PROGRAM MAIN
VAR
	//  8_Slave  and 248Input word /248Output word
	wArrScanner2AdapterInput_1				AT%I*		:ARRAY[0..247] OF WORD;
	wArrAdapter2ScannerOutput_1				AT%Q*		:ARRAY[0..247] OF WORD;
	wArrScanner2AdapterInput_2				AT%I*		:ARRAY[0..247] OF WORD;
	wArrAdapter2ScannerOutput_2				AT%Q*		:ARRAY[0..247] OF WORD;
	wArrScanner2AdapterInput_3				AT%I*		:ARRAY[0..247] OF WORD;
	wArrAdapter2ScannerOutput_3				AT%Q*		:ARRAY[0..247] OF WORD;
	wArrScanner2AdapterInput_4				AT%I*		:ARRAY[0..247] OF WORD;
	wArrAdapter2ScannerOutput_4				AT%Q*		:ARRAY[0..247] OF WORD;
	wArrScanner2AdapterInput_5				AT%I*		:ARRAY[0..247] OF WORD;
	wArrAdapter2ScannerOutput_5				AT%Q*		:ARRAY[0..247] OF WORD;
	wArrScanner2AdapterInput_6				AT%I*		:ARRAY[0..247] OF WORD;
	wArrAdapter2ScannerOutput_6				AT%Q*		:ARRAY[0..247] OF WORD;
	wArrScanner2AdapterInput_7				AT%I*		:ARRAY[0..247] OF WORD;
	wArrAdapter2ScannerOutput_7				AT%Q*		:ARRAY[0..247] OF WORD;
	wArrScanner2AdapterInput_8				AT%I*		:ARRAY[0..247] OF WORD;
	wArrAdapter2ScannerOutput_8				AT%Q*		:ARRAY[0..247] OF WORD;
	i,j			:INT;
END_VAR

FOR i :=0 TO 247 DO
	wArrAdapter2ScannerOutput_1[i]			:=i+1;
END_FOR


FOR j :=0 TO 247 DO
	wArrAdapter2ScannerOutput_8[j]			:=j+1;
END_FOR

END_PROGRAM
